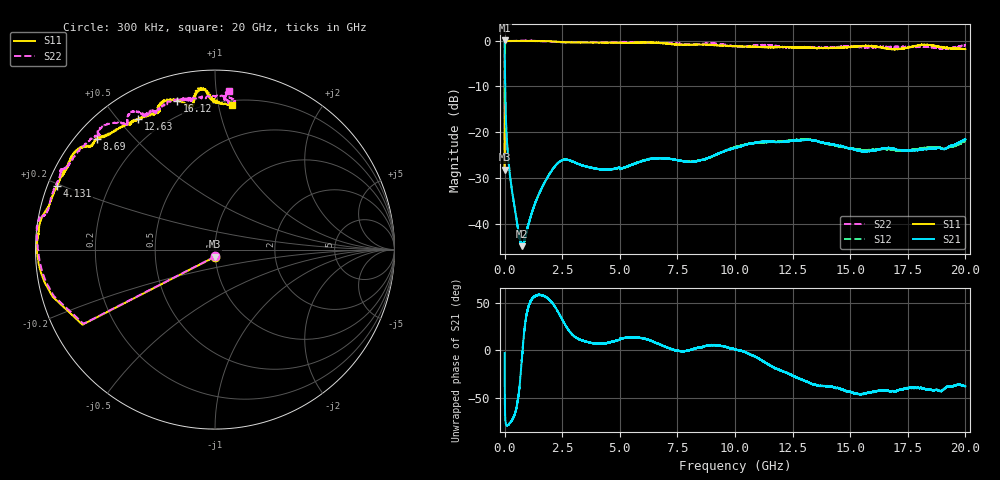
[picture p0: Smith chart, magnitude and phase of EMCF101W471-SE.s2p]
!EMCF101W471
!Johanson Technology Inc.
!www.johansontechnology.com
!Test Board Conditions:
!Substrate Type  RO4350B
!Substrate Thickness  6.6 mil
!Substrate Dk  3.66
!TL Type: GCPW
!TL Trace Width  13 mil
!TL Gap  7.5 mil
!PART MODE SINGLE ENDED (AKA BYPASS)
!DUT TOPOLOGY	SERIES-SHUNT
# MHz S  dB  R 50
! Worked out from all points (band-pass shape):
!   20001 points, 300 kHz to 20 GHz, reference 50 ohm
!   highest |S21| = 0.02 dB at 300 kHz (marker M1); lowest = -44.9 dB at 750.3 MHz (marker M2)
!   |S21| within 3 dB of the highest: start of sweep to 7.331 MHz
!   lowest |S11| = -28.2 dB at 300 kHz (marker M3), VSWR 1.08, Z = 50 - j3.9 ohm
!   |S11| at or under -10 dB: start of sweep to 2.58 MHz
!   |S22| runs from -28.4 to 0.0 dB; largest |S21 - S12| = 0.0047
!   S11 on the Smith chart (normalised r, x): 300 kHz: 1.00, -0.08; 4.131 GHz: 0.03, +0.19; 8.69 GHz: 0.06, +0.39; 12.63 GHz: 0.11, +0.57; 16.12 GHz: 0.13, +0.77; 20 GHz: 0.23, +1.09
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0.3  -28.18 -87.3  0.02 -2.7  0.02 -2.7  -28.43 -87.6
107.298  -0.11 -176.6  -22.44 -78.2  -22.40 -78.4  -0.19 -176.4
176.297  -0.09 -178.7  -26.70 -77.3  -26.69 -77.4  -0.13 -178.6
300.296  -0.06 179.5  -32.05 -73.7  -32.04 -73.8  -0.10 179.0
611.291  -0.07 176.8  -41.91 -45.7  -41.92 -45.6  -0.04 175.7
750.289  -0.08 175.9  -44.89 -9.2  -44.69 -9.1  -0.02 174.3
1427.279  -0.11 173.9  -34.21 57.8  -34.23 58.1  -0.09 169.5
2123.268  -0.20 168.8  -27.83 47.8  -27.78 47.6  -0.27 168.5
2603.261  -0.35 165.8  -26.00 27.9  -26.00 27.6  -0.38 166.8
3334.25  -0.40 162.5  -27.18 10.8  -27.18 10.7  -0.36 161.5
4131.238  -0.46 158.1  -28.12 7.0  -28.09 7.1  -0.41 156.4
6667.2  -0.50 143.5  -25.70 7.1  -25.66 6.9  -0.54 146.2
7864.182  -0.92 139.8  -26.44 -0.7  -26.38 -0.3  -0.76 135.9
8690.17  -0.90 136.8  -25.89 4.5  -25.94 4.3  -0.64 134.7
10000.15  -1.26 130.7  -23.45 1.1  -23.26 1.3  -1.30 125.8
12629.11  -1.46 120.4  -21.77 -28.0  -21.73 -27.4  -1.46 116.3
13334.1  -1.59 115.5  -21.78 -35.0  -21.69 -35.4  -1.53 113.8
16118.06  -1.37 104.4  -23.91 -42.5  -23.88 -44.4  -1.49 99.5
16667.05  -1.84 100.4  -23.44 -42.3  -23.74 -43.0  -1.39 101.8
17246.04  -1.75 98.5  -23.93 -40.8  -24.07 -39.5  -1.39 99.9
18606.02  -1.08 93.3  -23.58 -41.8  -23.35 -42.9  -1.52 83.2
20000  -1.82 83.5  -21.52 -37.5  -21.85 -36.1  -1.09 85.0
